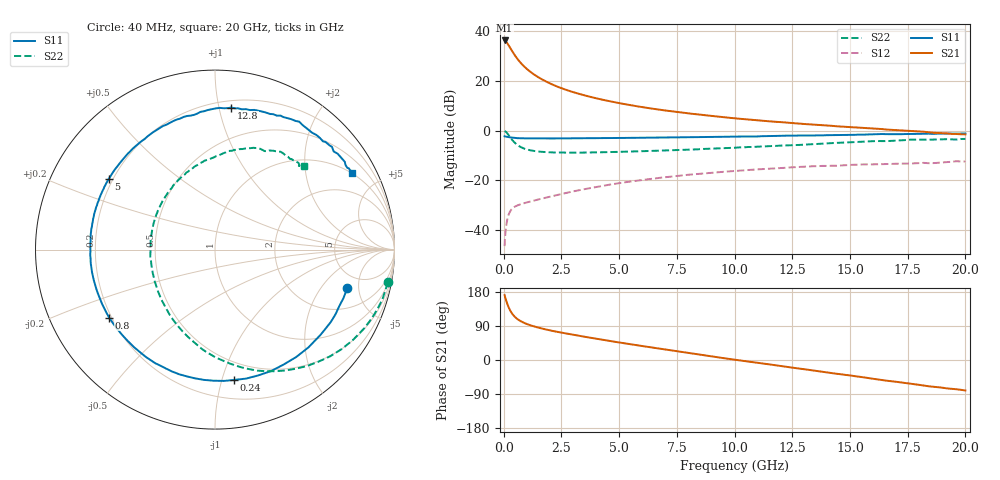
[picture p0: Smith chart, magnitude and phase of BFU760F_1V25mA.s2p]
! Filename:  P:\Prog\Test\Noise\ATS_data\Testdata_Net\Split files Spar\BFU760F_2W_C1_1V_5mA_60mA_Bias6_D.s2p
! Date/Time: Mon 06/Feb/2012 15:06:14
! BFU760_2W_C1_1V_5mA_60mA_Bias6_R.s2p
! MDIF S-parameter v. bias file
! BFU760_2W_C1_1V_5mA_60mA
! Date/time Fri Mar 18 10:56:44 2011
! VAR V_out= 1.0001
! VAR I_out= 24.9700
! VAR V_in= 0.7998
! VAR I_in= 0.0789
! Device data file deembeded for feedlines and parallel
! Original file: \Split files Spar\BFU760_2W_C1_1V_5mA_60mA_Bias6_R.s2p
! Feed-files: PR003V01_101208_Feed1.s2p, PR003V01_101208_Feed2.s2p
! Parallel-file: PR003V01_101208_Par.s2p
# MHz S MA R 50
!  Freq-MHz  S11-mag  S11-arg  S21-mag  S21-arg  S12-mag  S12-arg  S22-mag  S22-arg
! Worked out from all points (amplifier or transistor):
!   167 points, 40 MHz to 20 GHz, reference 50 ohm
!   highest |S21| = 36.3 dB at 40 MHz (marker M1)
!   |S21| within 3 dB of that: start of sweep to 281.6 MHz
!   unconditionally stable (mu >= 1): 3.91 GHz to 15.15 GHz
!   at 550 MHz: K = 0.30, MSG = 29.9 dB, |S12| = -30.3 dB
!   at 4.2 GHz: K = 1.01, MAG = 16.8 dB, |S12| = -22.4 dB
!   at 20 GHz: K = 0.94, MSG = 5.5 dB, |S12| = -12.4 dB
!   S11 on the Smith chart (normalised r, x): 40 MHz: 3.56, -3.73; 240 MHz: 0.35, -1.10; 800 MHz: 0.19, -0.28; 5 GHz: 0.18, +0.29; 12.8 GHz: 0.25, +1.09; 20 GHz: 0.99, +3.59
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40  0.7678 -16.3  65.38 171.3  0.004704 83.2  0.9799 -10.7
50  0.765 -20.8  64.92 168.4  0.006172 77.4  0.9754 -13.8
60  0.7607 -24.4  63.51 166.4  0.006882 77.7  0.9729 -16.6
90  0.7571 -35.8  62.63 160.2  0.0102 74.0  0.9493 -25.0
140  0.7502 -52.9  58.8 150.9  0.01489 66.4  0.8982 -38.0
180  0.7452 -65.2  55.27 144.4  0.01807 61.0  0.8496 -47.4
240  0.7341 -81.6  49.9 135.7  0.02175 54.4  0.7791 -59.8
340  0.7236 -102.5  41.73 124.7  0.0259 46.6  0.6746 -77.0
460  0.7126 -120.3  34.09 115.3  0.02895 41.1  0.5833 -92.7
600  0.7037 -134.2  27.61 107.8  0.03122 37.8  0.5105 -106.8
800  0.7007 -147.3  21.5 100.4  0.03367 35.7  0.452 -121.9
1200  0.6962 -163.0  14.73 90.8  0.03783 36.0  0.3971 -142.0
1700  0.6957 -174.7  10.51 82.4  0.04327 37.9  0.3718 -157.7
2400  0.6962 174.5  7.446 73.4  0.05155 39.8  0.3619 -172.3
3400  0.7016 162.5  5.277 62.5  0.0649 39.8  0.3617 173.3
5000  0.7106 146.5  3.579 46.3  0.08734 35.6  0.3733 155.2
6800  0.7232 130.8  2.62 29.5  0.1124 27.6  0.3955 138.5
10200  0.7595 103.3  1.736 -0.8  0.1562 8.1  0.4582 110.3
12800  0.7963 83.5  1.386 -22.5  0.1858 -8.2  0.5145 90.5
13400  0.7958 79.1  1.321 -27.6  0.1915 -12.9  0.5319 86.4
16800  0.8475 53.5  1.033 -56.0  0.2132 -34.6  0.6215 62.0
20000  0.8746 29.2  0.8415 -80.5  0.239 -55.8  0.6801 43.3
